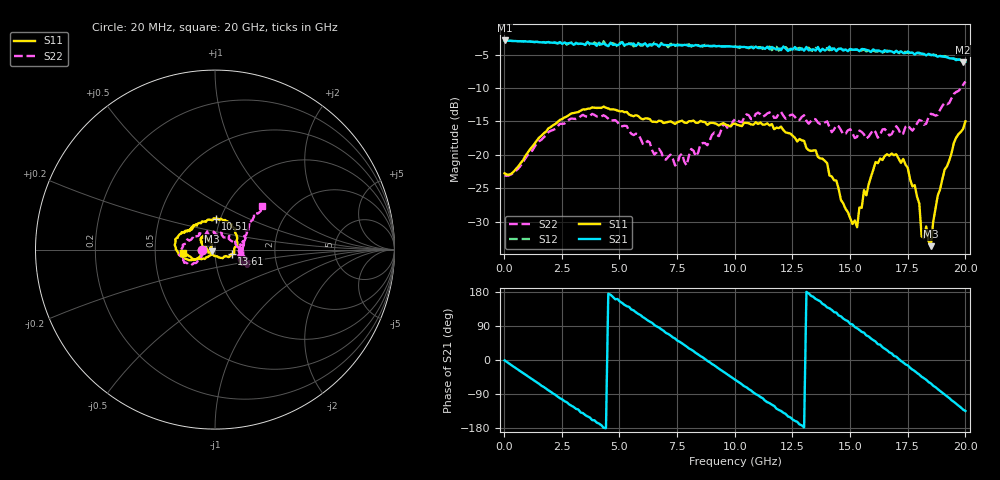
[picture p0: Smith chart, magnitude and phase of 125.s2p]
!Agilent Technologies,N5230A,US43500223,A.07.50.48
!Agilent N5230A: A.07.50.48
!Date: Wednesday, September 16, 2015 18:24:23
!Correction: S11(Full 2 Port(1,2))
!S21(Full 2 Port(1,2))
!S12(Full 2 Port(1,2))
!S22(Full 2 Port(1,2))
!S2P File: Measurements: S11, S21, S12, S22:
# Hz S  dB  R 50
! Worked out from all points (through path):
!   201 points, 20 MHz to 20 GHz, reference 50 ohm
!   highest |S21| = -2.89 dB at 20 MHz (marker M1); lowest = -6.1 dB at 19.9 GHz (marker M2)
!   group delay of S21, straight-line fit = 117 ps
!   lowest |S11| = -33.7 dB at 18.5 GHz (marker M3), VSWR 1.04, Z = 48.2 - j0.858 ohm
!   |S11| at or under -10 dB: start of sweep to end of sweep
!   |S22| runs from -23.1 to -9.0 dB; largest |S21 - S12| = 0.041
!   S11 on the Smith chart (normalised r, x): 20 MHz: 0.86, -0.00; 10.51 GHz: 0.95, +0.34; 13.61 GHz: 1.20, -0.06; 20 GHz: 0.70, -0.03
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2e7  -22.77 -179.7  -2.89 -0.9  -2.89 -0.9  -23.11 179.7
1.9181e9  -16.04 -158.1  -3.13 -80.0  -3.13 -80.4  -16.61 -146.9
3.4166e9  -13.21 179.4  -3.40 -140.1  -3.71 -139.4  -14.03 -163.9
4.3157e9  -12.79 165.6  -3.34 -178.9  -3.01 -177.1  -14.08 -180.0
5.1149e9  -13.47 155.6  -3.14 150.7  -3.11 150.5  -15.72 163.4
6.7133e9  -14.90 141.5  -3.79 85.8  -3.82 85.0  -19.10 113.1
8.3117e9  -15.20 131.9  -3.56 18.6  -3.55 20.1  -20.25 38.1
1.001e10  -15.34 102.8  -3.82 -51.7  -3.81 -52.1  -14.65 -14.7
1.05095e10  -15.23 88.7  -3.92 -72.2  -3.96 -73.1  -13.94 -18.5
1.22078e10  -16.65 40.3  -4.13 -142.3  -3.90 -145.6  -14.60 -24.4
1.34066e10  -19.36 -4.9  -4.20 166.7  -4.48 166.8  -14.61 -31.2
1.36064e10  -20.33 -14.9  -3.86 158.0  -4.07 156.7  -15.19 -23.5
1.53047e10  -30.84 -150.7  -4.23 83.7  -4.26 83.2  -17.31 -14.7
1.61039e10  -21.08 152.3  -4.42 48.8  -4.55 48.4  -16.60 2.6
1.67033e10  -20.12 138.2  -4.45 20.1  -4.53 20.5  -17.09 9.5
1.75025e10  -21.95 125.6  -4.54 -14.1  -4.74 -15.8  -15.56 13.4
1.8002e10  -27.30 118.7  -4.74 -38.4  -4.84 -38.6  -14.78 20.8
1.81019e10  -32.21 132.8  -4.91 -44.2  -4.84 -43.7  -14.93 25.4
1.85015e10  -33.67 -154.5  -5.05 -61.7  -5.10 -62.8  -13.86 28.3
1.91009e10  -22.22 -137.6  -5.34 -91.0  -5.23 -92.0  -12.23 38.5
1.99001e10  -16.14 -169.3  -6.14 -131.0  -6.03 -133.1  -9.54 40.2
2e10  -15.00 -174.2  -6.06 -134.6  -6.24 -137.5  -9.03 42.8
